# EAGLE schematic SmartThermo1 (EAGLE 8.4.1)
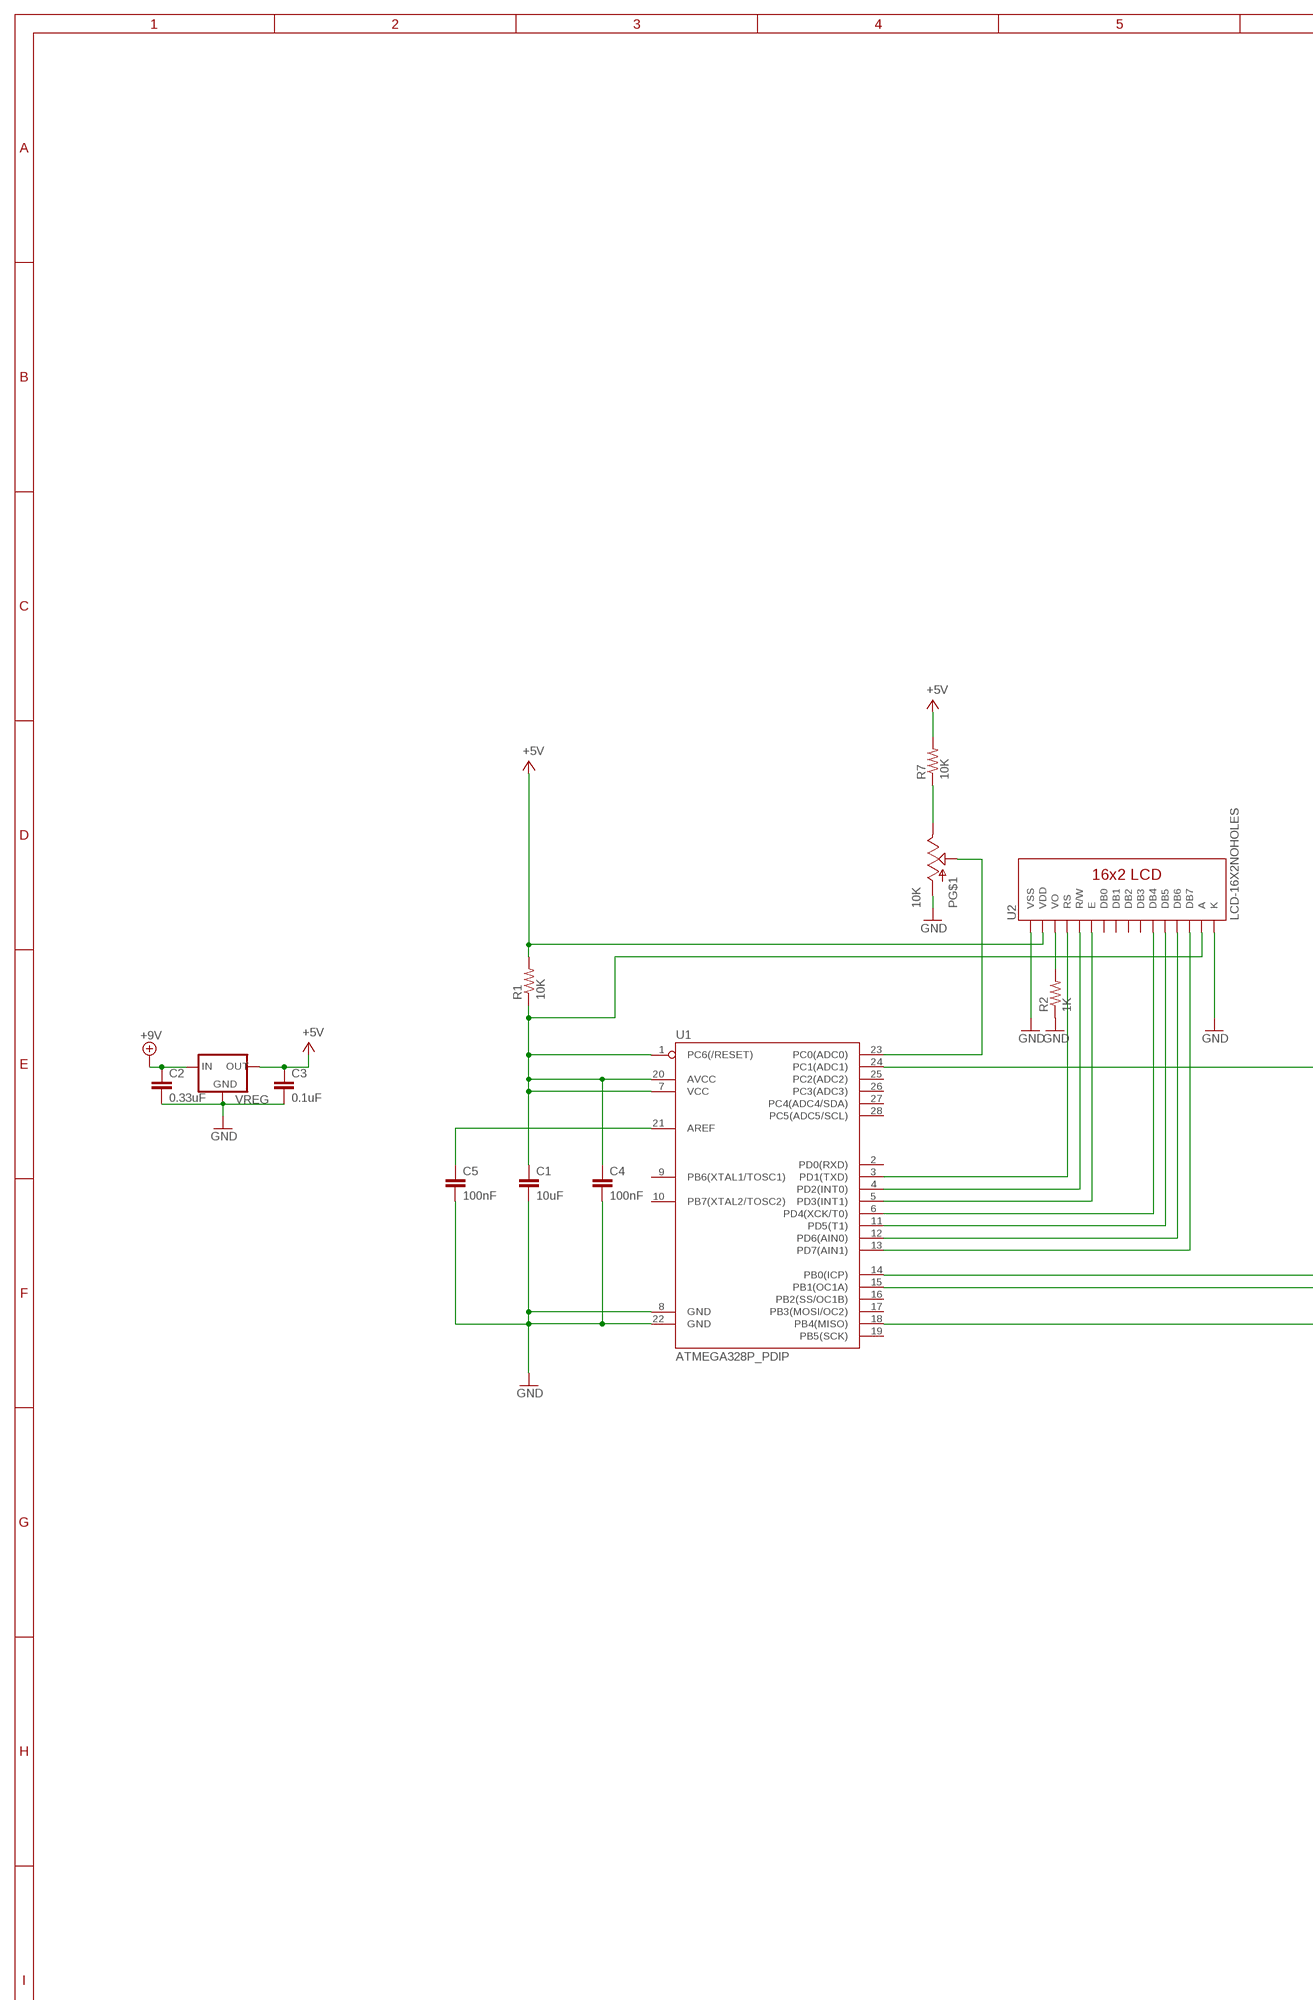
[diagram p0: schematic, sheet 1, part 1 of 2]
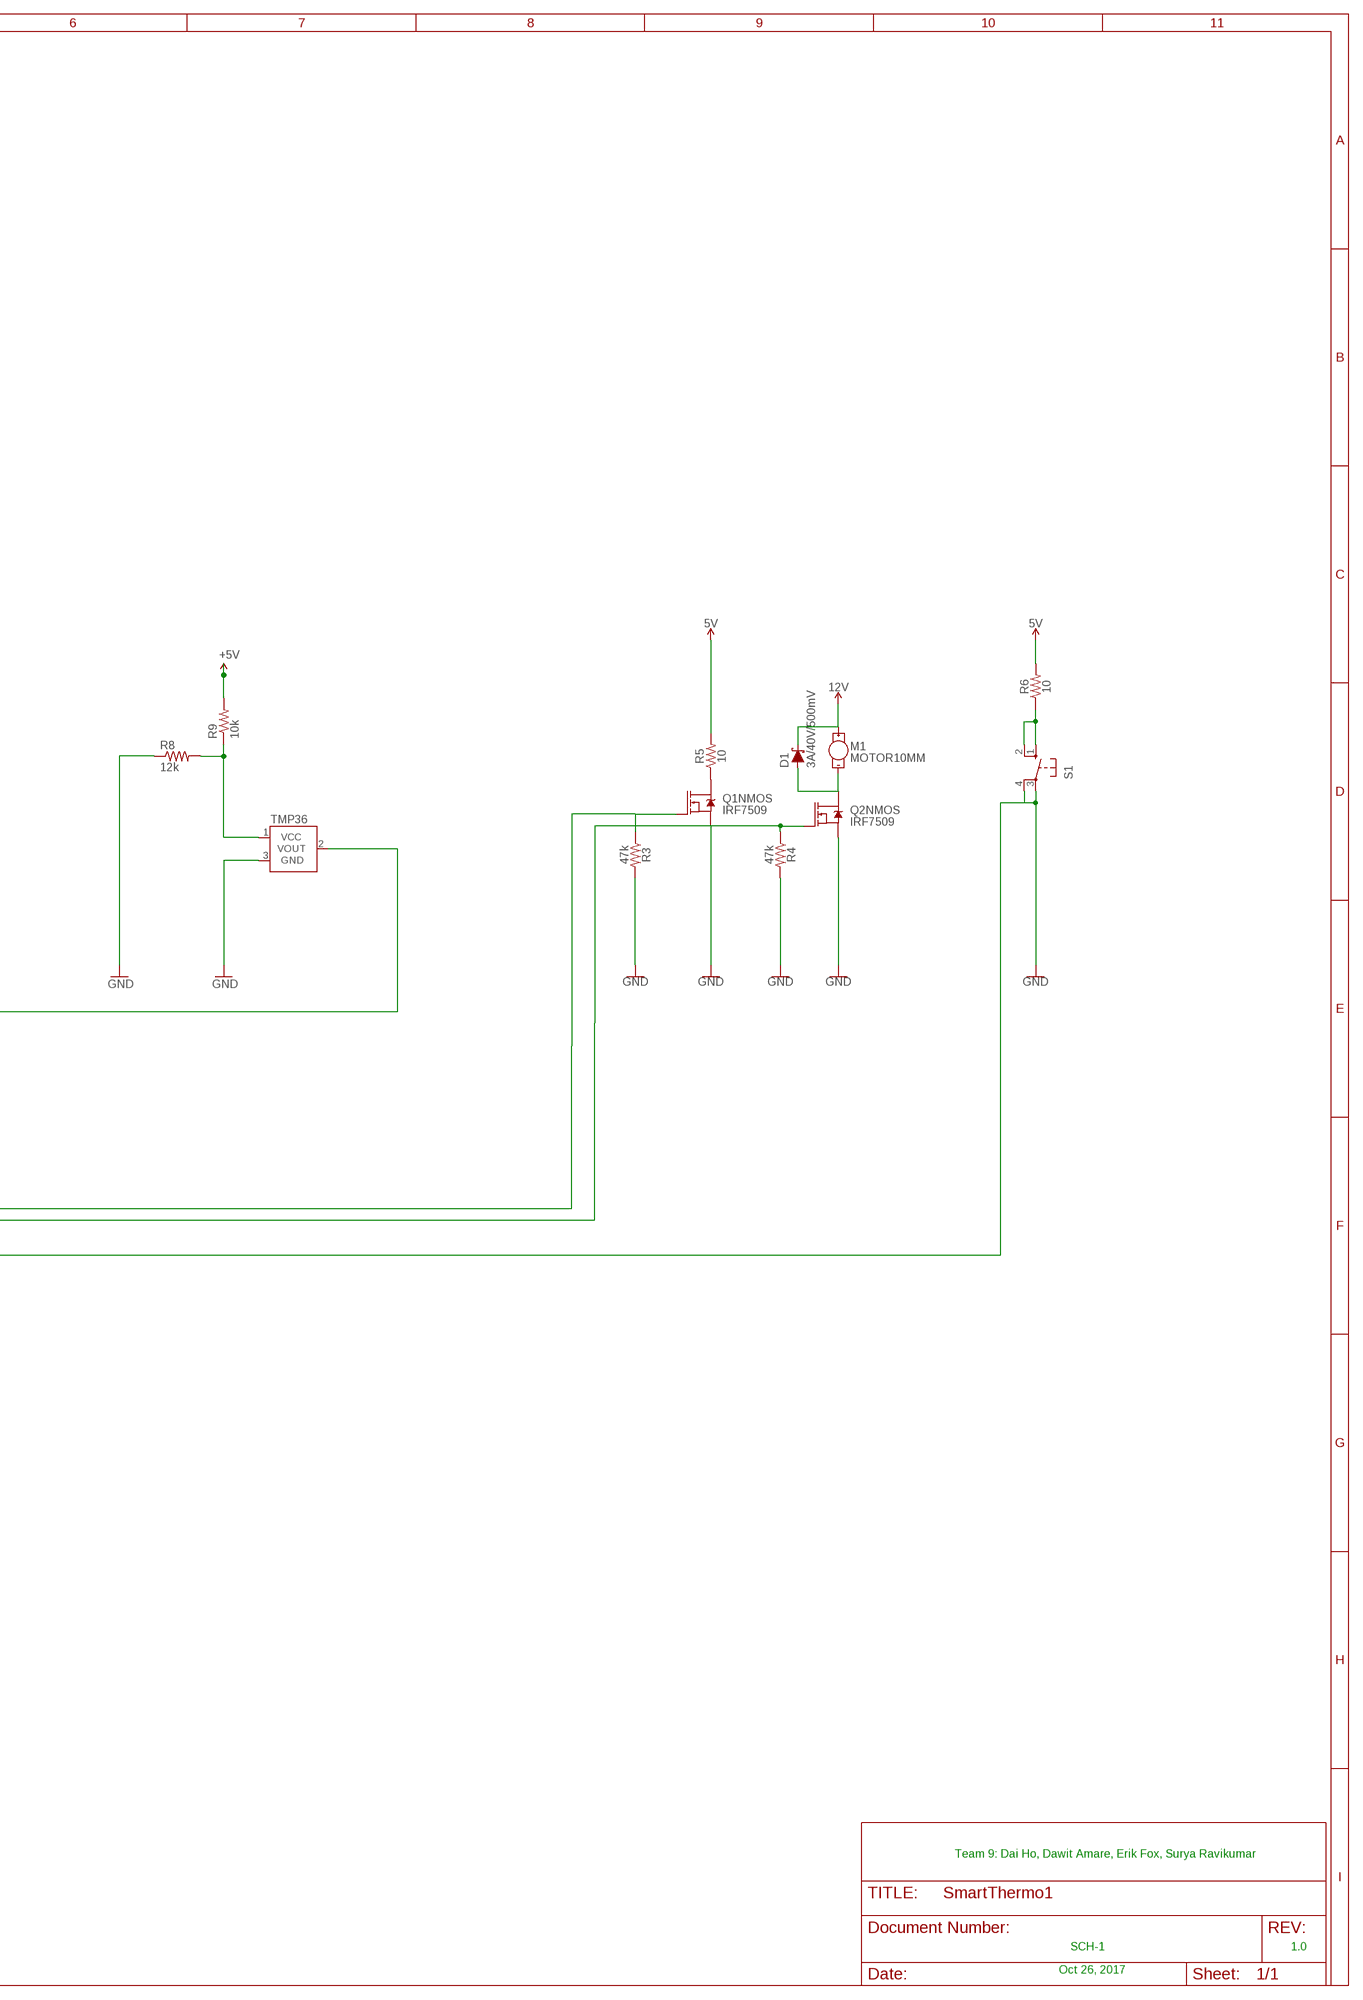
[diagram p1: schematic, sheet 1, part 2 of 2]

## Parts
C1  10uF  10UF-6.3V-20%(1206)  [1206]
C2  0.33uF  C7.5/3  [C7.5B3]
C3  0.1uF  C7.5/3  [C7.5B3]
C4  100nF  C2.5/2  [C2.5-2]
C5  100nF  C2.5/2  [C2.5-2]
D1  3A/40V/500mV  DIODE-SCHOTTKY-B340A  [SMA-DIODE]
M1  MOTOR10MM  [VIBE-MOTOR-10MM]
P  10K  POT_SWITCHPOT_PTH  [POT_PTH]
Q1  IRF7509  [MSOP8]
Q2  IRF7509  [MSOP8]
R1  10K  RESISTOR1206  [1206]
R2  1K  1KOHM1/10W1%(0603)  [0603-RES]
R3  47k  47KOHM-0603-1/10W-1%  [0603]
R4  47k  47KOHM-0603-1/10W-1%  [0603]
R5  10  10OHM-0603-1/10W-5%  [0603]
R6  10  10OHM-0603-1/10W-5%  [0603]
R7  10K  RESISTOR1206  [1206]
R8  12k  R-US_0207/5V  [0207/5V]
R9  10k  R-US_0207/5V  [0207/5V]
S1  10-XX  [B3F-10XX]
TMP36  TMP36GT9  [TO-92]
U1  ATMEGA328P_PDIP  [DIL28-3]
U2  LCD-16X2NOHOLES  [LCD-16X2_NOHOLES]
VREG  V_REG_78XX-TO-220  [TO-220-ALT]

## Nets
5V: R5.2 R6.2
12V: D1.C M1.+
+9V: C2.1 VREG.IN
GND: C1.2 C2.2 C3.2 C4.2 C5.2 P.E@1(A) Q1.1(NMOS:S) Q2.1(NMOS:S) R2.1 R3.2 R4.2 R8.1 S1.3(P) S1.4(P1) TMP36.3(GND) U1.8(GND) U1.18(PB4(MISO)) U1.22(GND) U2.1(VSS) U2.16(K) VREG.GND
N$1: C1.1 C4.1 R1.1 U1.1(PC6(/RESET)) U1.7(VCC) U1.20(AVCC) U2.15(A)
N$2: TMP36.2(VOUT) U1.24(PC1(ADC1))
N$3: Q1.2(NMOS:G) R3.1 U1.14(PB0(ICP))
N$4: Q2.2(NMOS:G) R4.1 U1.15(PB1(OC1A))
N$5: U1.3(PD1(TXD)) U2.4(RS)
N$6: U1.4(PD2(INT0)) U2.5(R/W)
N$7: U1.5(PD3(INT1)) U2.6(E)
N$8: U1.6(PD4(XCK/T0)) U2.11(DB4)
N$9: U1.11(PD5(T1)) U2.12(DB5)
N$10: U1.12(PD6(AIN0)) U2.13(DB6)
N$11: U1.13(PD7(AIN1)) U2.14(DB7)
N$12: R8.2 R9.1 TMP36.1(VCC)
N$13: D1.A M1.- Q2.7(NMOS:D) Q2.8(NMOS:D)
N$14: Q1.7(NMOS:D) Q1.8(NMOS:D) R5.1
N$15: R6.1 S1.1(S) S1.2(S1)
N$16: R2.2 U2.3(VO)
N$17: P.E@2(E) R7.1
N$18: P.WAND(S) U1.23(PC0(ADC0))
N$19: C5.1 U1.21(AREF)
V+: C3.1 R1.2 R7.2 U2.2(VDD) VREG.OUT ; supply symbol labelled +5V
VCC: R9.2 ; supply symbol labelled +5V
Unconnected: P.S1 P.S2 Q1.3(PMOS:S) Q1.4(PMOS:G) Q1.5(PMOS:D) Q1.6(PMOS:D) Q2.3(PMOS:S) Q2.4(PMOS:G) Q2.5(PMOS:D) Q2.6(PMOS:D) U1.2(PD0(RXD)) U1.9(PB6(XTAL1/TOSC1)) U1.10(PB7(XTAL2/TOSC2)) U1.16(PB2(SS/OC1B)) U1.17(PB3(MOSI/OC2)) U1.19(PB5(SCK)) U1.25(PC2(ADC2)) U1.26(PC3(ADC3)) U1.27(PC4(ADC4/SDA)) U1.28(PC5(ADC5/SCL)) U2.7(DB0) U2.8(DB1) U2.9(DB2) U2.10(DB3)

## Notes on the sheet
- Team 9: Dai Ho, Dawit Amare, Erik Fox, Surya Ravikumar
- SCH-1 | 1.0
- Oct 26, 2017

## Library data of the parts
C1 = SparkFun-Capacitors:10UF-6.3V-20%(1206): CAP-10057; PROD_ID: CAP-10057
C2-C5 = capacitor-wima:C: CAPACITOR
D1 = SparkFun-DiscreteSemi:DIODE-SCHOTTKY: Schottky diode; PROD_ID: DIO-09886
M1 = SparkFun-Electromechanical:MOTOR: Motor (Single-Phase); PROD_ID: COMP-08572; SF_SKU: ROB-08449
P = button_TestFootprint:POT_SWITCH: Potentiometer w/ switch.
Q1 Q2 = SparkFun-DiscreteSemi:IRF7509: Dual N and P Channel MOSFET Dual N/P-Channel 30V 1.25 W 7.8/7.5 nC Hexfet Power Mosfet Surface Mount-MICRO-8. NMOS RDS(ON) 0.11Ω. PMOS RDS(ON) 0.20Ω. Link to datasheet SparkFun Products: SparkFun RedBot Mainboard SparkFun Wake on Shake; PROD_ID: TRANS-07913
R1 R7 = SparkFun-Passives:RESISTOR: Resistor
R2 = SparkFun-Resistors:1KOHM1/10W1%(0603): RES-07856; PROD_ID: RES-07856
R3 R4 = SparkFun-Resistors:47KOHM: 47kΩ resistor; PROD_ID: RES-07871
R5 R6 = SparkFun-Resistors:10OHM: 10Ω resistor; PROD_ID: RES-09834
R8 R9 = resistor:R-US_: RESISTOR, American symbol
S1 = switch-omron:10-XX: OMRON SWITCH; MPN: B3F-1000; OC_FARNELL: 176432; OC_NEWARK: 36M3542
TMP36 = SparkFun-Sensors:TMP36: Precision degC temp sensor, analog out
U1 = SparkFun-DigitalIC:ATMEGA328P_PDIP: uC used in the Arduino 32kb flash, 1k EEPROM, 2k SRAM This is the through-hole version of this chip.
U2 = SparkFun-Displays:LCD-16X2: Standard text-only 16x2 parallel input LCD
VREG = SparkFun-PowerIC:V_REG_78XX: Voltage Regulator Standard 7805 5V regulator. IGO (Input Ground Output). Spark Fun Electronics SKU : COM-00107

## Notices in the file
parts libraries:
SparkFun-DigitalIC: Licensing: Creative Commons ShareAlike 4.0 International - https://creativecommons.org/licenses/by-sa/4.0
